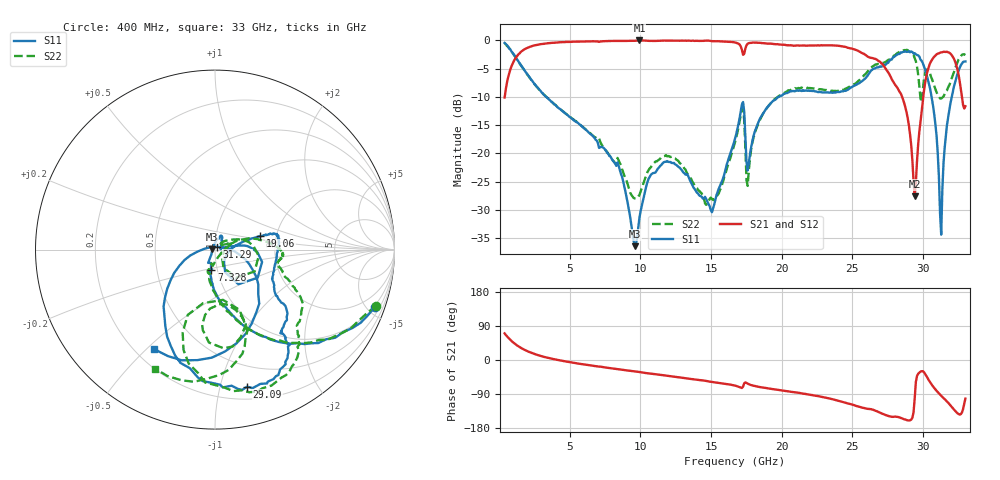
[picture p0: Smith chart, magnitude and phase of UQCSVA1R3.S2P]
!  Part Number  UQCSVA1R3  Mounting Orientation: Horizontal
!  Description: Ultra Low ESR Microwave capacitors
!  Application: Coupling, Bypass, Tuning, DC Block
!  Filters, Matching
# GHZ S DB R 50
! Freq  |S11|  S11 Ph  |S21|  S21 Ph  |S12|  S12 Ph  |S22|  S22 Ph
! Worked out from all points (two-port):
!   401 points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, 400 MHz to 33 GHz, reference 50 ohm
!   highest |S21| = -0.02 dB at 9.936 GHz (marker M1); lowest = -27.6 dB at 29.41 GHz (marker M2)
!   |S21| within 3 dB of the highest: 1.22 GHz to 26.21 GHz (24.99 GHz wide, 182 % of centre); 30.76 GHz to 32.13 GHz (1.375 GHz wide, 4.37 % of centre)
!   lowest |S11| = -36.4 dB at 9.61 GHz (marker M3), VSWR 1.03, Z = 48.5 + j0.082 ohm
!   |S11| at or under -10 dB: 3.347 GHz to 19.81 GHz (16.46 GHz wide, 142 % of centre); 30.61 GHz to 32.04 GHz (1.431 GHz wide, 4.57 % of centre)
!   |S22| runs from -29.1 to -0.5 dB; largest |S21 - S12| = 0.0091
!   S11 on the Smith chart (normalised r, x): 400 MHz: 0.90, -5.66; 7.328 GHz: 0.94, -0.21; 19.06 GHz: 1.64, +0.26; 29.09 GHz: 0.31, -1.22; 31.29 GHz: 1.02, +0.03; 33 GHz: 0.28, -0.53
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0.4  -0.46 -19.6  -10.11 70.2  -10.12 70.1  -0.45 -19.2
2.275  -6.93 -69.5  -1.07 19.1  -1.06 19.2  -6.96 -69.8
5.861  -15.22 -96.7  -0.22 -10.9  -0.22 -10.9  -15.17 -100.1
7.328  -18.94 -100.4  -0.16 -18.6  -0.16 -18.6  -18.70 -107.1
8.55  -22.93 -118.2  -0.12 -25.1  -0.12 -25.2  -21.66 -95.4
9.61  -36.43 176.8  -0.08 -30.0  -0.09 -30.1  -27.98 -40.8
9.936  -31.46 109.4  -0.02 -31.8  -0.04 -31.9  -27.38 -13.7
11.321  -22.51 70.6  -0.06 -38.6  -0.08 -38.8  -21.09 19.6
15.07  -30.42 9.8  -0.14 -57.8  -0.14 -57.7  -28.06 43.6
16.7  -17.42 9.7  -0.36 -67.7  -0.36 -67.5  -18.07 26.8
17.189  -11.33 -14.7  -1.66 -73.9  -1.66 -73.6  -12.18 -8.4
17.678  -21.73 -4.1  -0.50 -63.9  -0.50 -64.0  -23.05 13.0
19.064  -11.66 16.7  -0.59 -75.0  -0.56 -74.9  -11.60 11.6
22.161  -8.98 4.4  -0.93 -92.5  -0.91 -92.4  -8.48 -6.0
27.621  -3.63 -52.3  -6.01 -148.6  -6.04 -148.8  -3.40 -46.9
29.088  -2.11 -76.8  -16.74 -159.1  -16.67 -158.5  -1.99 -82.6
29.414  -2.28 -86.7  -27.62 -100.9  -27.24 -100.0  -3.16 -97.7
29.822  -3.41 -102.0  -14.47 -30.6  -14.37 -31.3  -10.28 -102.6
30.555  -9.24 -140.6  -3.78 -61.4  -3.84 -61.3  -6.36 -96.3
31.289  -34.39 56.0  -2.12 -94.3  -2.17 -94.0  -10.30 -83.2
32.267  -7.50 -57.2  -3.72 -133.8  -3.75 -134.0  -5.00 -72.9
33  -3.74 -121.2  -11.67 -101.9  -11.49 -102.3  -2.59 -116.6
